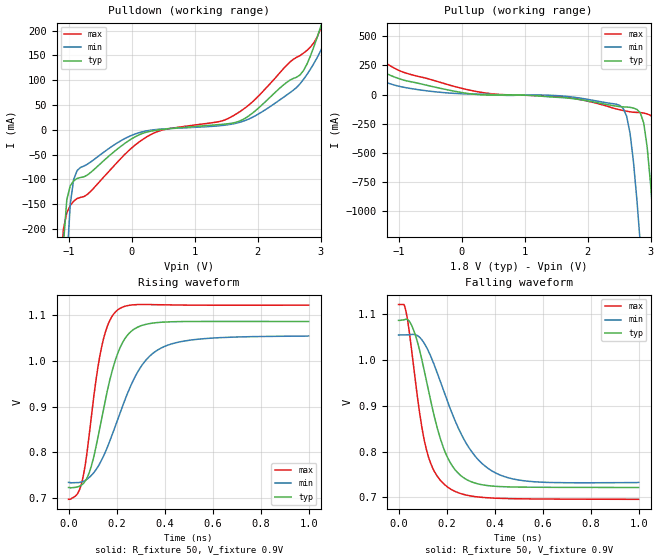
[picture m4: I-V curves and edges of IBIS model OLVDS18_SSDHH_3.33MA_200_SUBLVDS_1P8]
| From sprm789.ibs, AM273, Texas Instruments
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|   Model Cell OLVDS18_SSDHH_3.33MA_200_SUBLVDS_1P8
|OLVDS18_SSDHH_3.33MA_200_SUBLVDS_1P8
[Model]   OLVDS18_SSDHH_3.33MA_200_SUBLVDS_1P8
Model_type   Output
Polarity   Non-Inverting
Cref =  15.0001pF
Rref =  101.0000M
Vref =  0V
Vmeas =  1.08
C_comp   1.5p   1.5p   1.5p
[Temperature Range]   25   125   -40
[Voltage Range]   1.8   1.62   1.98
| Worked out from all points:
|   slope of the pulldown table from 0 to 0.27 V, typ, clamps not added: 18.9 ohm
|   slope of the pullup table from 0 to 0.27 V, typ, clamps not added: 15 ohm
|   rising waveform, R_fixture 50, V_fixture 0.9V: 20-80 % time 95.3ps typ, 154ps min, 68.1ps max; typ from 0.722 V to 1.09 V
|   falling waveform, R_fixture 50, V_fixture 0.9V: 20-80 % time 106ps typ, 160ps min, 78.2ps max; typ from 1.09 V to 0.721 V
| Nom Voltages:
|   BIAS1=1.2, BIAS2=1.2, VDD=1.1, VDDS=1.8, BUS_BIAS3=0, BUS_VSSS=0,
|   ESD_BIASFET=0, VSS=0
| Min Voltages:
|   BIAS1=1.2, BIAS2=1.2, VDD=0.99, VDDS=1.62, BUS_BIAS3=0, BUS_VSSS=0,
|   ESD_BIASFET=0, VSS=0
| Max Voltages:
|   BIAS1=1.2, BIAS2=1.2, VDD=1.21, VDDS=1.98, BUS_BIAS3=0, BUS_VSSS=0,
|   ESD_BIASFET=0, VSS=0
[Pulldown]
|   voltage   I(typ)   I(min)   I(max)
-1.8V     -5.997A    -6.311A    -5.864A
-1.091V   -231.8mA   -488.8mA   -200.9mA
-1.036V   -141.1mA   -270.2mA   -167.6mA
-927.3mV  -103mA     -100.2mA   -144.1mA
-872.7mV  -98.29mA   -82.32mA   -138.7mA
-218.2mV  -37.51mA   -25.32mA   -63.46mA
381.8mV   -1.063mA   384.4uA    -4.836mA
1.909V    32.8mA     24.69mA    55.41mA
2.727V    119.3mA    101.5mA    154.4mA
3V        207.6mA    159.2mA    203.7mA
3.109V    251.8mA    227.9mA    251.8mA
3.6V      479.8mA    839mA      532mA
[Pullup]
|   voltage   I(typ)   I(min)   I(max)
-1.8V     414.4mA    369.7mA    571.9mA
-1.418V   253.3mA    146.7mA    359.8mA
-872.7mV  116.5mA    56.94mA    181.3mA
2.509V    -104mA     -93.54mA   -130.9mA
2.673V    -110.3mA   -333.5mA   -148.8mA
2.782V    -128.3mA   -906.1mA   -154mA
2.836V    -158mA     -1.288A    -155.5mA
2.945V    -454.5mA   -2.149A    -167.2mA
3.055V    -1.167A    -3.082A    -203.8mA
3.164V    -2.058A    -4.046A    -493.9mA
3.273V    -3.02A     -5.011A    -1.258A
3.6V      -6A        -7.905A    -4.194A
[Ramp]
| variable   typ   min   max
dV/dt_f 0.12637325/0.11649453n 0.10739797/0.15411119n 0.17058899/0.1266705n
dV/dt_r 0.18570541/92.684095p 0.13995013/0.14217945n 0.24681861/70.305874p
R_load = 50
[Rising Waveform]
R_fixture = 50
V_fixture = 0.9V
V_fixture_min = 0.9V
V_fixture_max = 0.9V
|   time   V(typ)   V(min)   V(max)
0s        722.3mV    733.6mV    696.3mV
50.19ps   726.5mV    733.8mV    724mV
87.05ps   756.1mV    744.8mV    842mV
113.6ps   809.6mV    760.8mV    955.4mV
140.4ps   880.5mV    785.2mV    1.037V
170.1ps   954.2mV    821.7mV    1.087V
202.1ps   1.013V     867.7mV    1.111V
293.8ps   1.076V     981.2mV    1.124V
398.4ps   1.086V     1.032V     1.123V
1ns       1.087V     1.055V     1.123V
[Falling Waveform]
R_fixture = 50
V_fixture = 0.9V
V_fixture_min = 0.9V
V_fixture_max = 0.9V
|   time   V(typ)   V(min)   V(max)
0s        1.087V     1.055V     1.121V
22.5ps    1.087V     1.055V     1.121V
33.7ps    1.089V     1.055V     1.099V
71.96ps   1.051V     1.055V     946.6mV
116ps     954.9mV    1.028V     804.4mV
148.5ps   877.7mV    989.5mV    757.3mV
198.6ps   793.4mV    917mV      724.8mV
304.4ps   733.7mV    799.9mV    702.7mV
419ps     723.6mV    749.7mV    697.9mV
1ns       721.5mV    732.7mV    695.7mV
